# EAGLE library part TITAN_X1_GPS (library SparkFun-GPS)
Titan X1 GPS
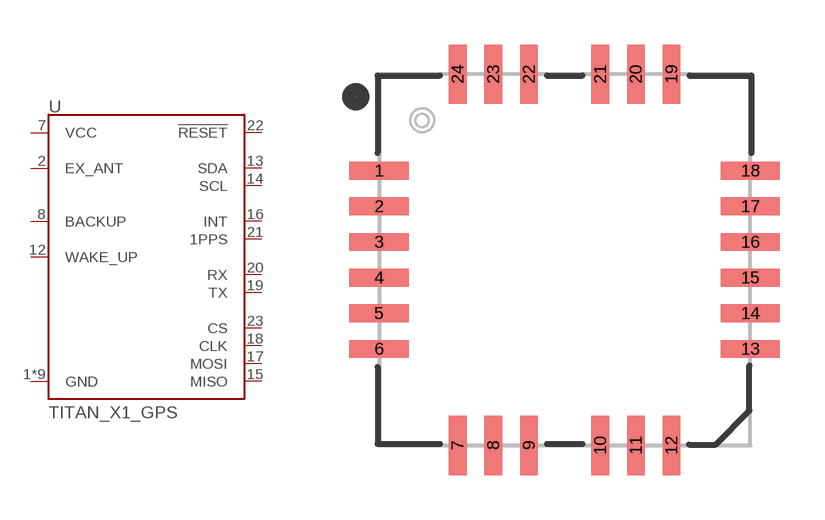
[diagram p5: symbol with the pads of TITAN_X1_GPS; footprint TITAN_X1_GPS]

Designator prefix U

## TITAN_X1_GPS (PROD_ID: GPS-13693; VALUE: Titan X1 GPS)  [TITAN_X1_GPS]
1  GND
2  EX_ANT
3  GND
4  GND
5  GND
6  GND
7  VCC
8  BACKUP
9  GND
10  GND
11  GND
12  WAKE_UP
13  SDA
14  SCL
15  MISO
16  INT
17  MOSI
18  CLK
19  TX
20  RX
21  1PPS
22  !RESET
23  CS
24  GND

## Footprint TITAN_X1_GPS (pad centres in mm)
smd 2 x 0.6: 1 -6.25,3; 2 -6.25,1.8; 3 -6.25,0.6; 4 -6.25,-0.6; 5 -6.25,-1.8; 6 -6.25,-3; 13 6.25,-3; 14 6.25,-1.8; 15 6.25,-0.6; 16 6.25,0.6; 17 6.25,1.8; 18 6.25,3
smd 0.6 x 2: 7 -3.6,-6.25; 8 -2.4,-6.25; 9 -1.2,-6.25; 10 1.2,-6.25; 11 2.4,-6.25; 12 3.6,-6.25; 19 3.6,6.25; 20 2.4,6.25; 21 1.2,6.25; 22 -1.2,6.25; 23 -2.4,6.25; 24 -3.6,6.25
